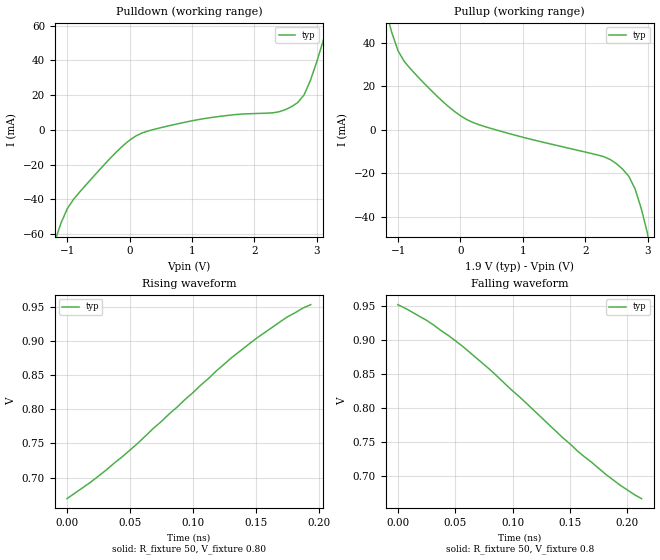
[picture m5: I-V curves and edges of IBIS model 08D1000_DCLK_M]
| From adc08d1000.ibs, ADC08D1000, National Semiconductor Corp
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[Model]   08D1000_DCLK_M
Model_type Output
Polarity Inverting
Vref=0.80
Vmeas=0.80
Rref=50   | 100 Ohms Across Outputs OUTP and OUTM
Cref=5p
|   TYP   MIN   MAX
C_comp   1.5p   1.5p   1.5p
[Temperature Range] 25   85   -40
[Voltage Range]   1.90   1.80   2.00
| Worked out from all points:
|   slope of the pulldown table from 0 to 0.285 V, typ, clamps not added: 55.2 ohm
|   slope of the pullup table from 0 to 0.285 V, typ, clamps not added: 71.5 ohm
|   falling waveform, R_fixture 50, V_fixture 0.8: 20-80 % time 113ps typ, NA min, NA max; typ from 0.952 V to 0.666 V
|   rising waveform, R_fixture 50, V_fixture 0.80: 20-80 % time 104ps typ, NA min, NA max; typ from 0.669 V to 0.953 V
[Pullup]
|Vtable   I(typ)   I(min)   I(max)
-1.9V     495.4mA    NA         NA
-1.2V     54.99mA    NA         NA
-1.1V     44.5mA     NA         NA
-1V       36.18mA    NA         NA
-800mV    27.93mA    NA         NA
-300mV    13.4mA     NA         NA
100mV     4.739mA    NA         NA
2.5V      -15.49mA   NA         NA
2.7V      -21.31mA   NA         NA
2.8V      -27.03mA   NA         NA
3V        -47.49mA   NA         NA
3.8V      -638.1mA   NA         NA
[Pulldown]
|V(pulldown)   I(typ)   I(min)   I(max)
-1.9V     -644.8mA   NA         NA
-1.2V     -64.35mA   NA         NA
-1V       -45.47mA   NA         NA
-800mV    -35.81mA   NA         NA
-200mV    -12.33mA   NA         NA
200mV     -1.805mA   NA         NA
1.1V      5.884mA    NA         NA
2.3V      9.828mA    NA         NA
2.6V      13.43mA    NA         NA
2.8V      20.25mA    NA         NA
3.2V      63.31mA    NA         NA
3.8V      497.3mA    NA         NA
[Ramp]
|   TYP   MIN   MAX
dV/dt_r   164mv/.096ns   NA   NA
dV/dt_f   164mv/.105ns   NA   NA
R_load=50
[Falling Waveform]
R_fixture=50
V_fixture=0.8
|Time   V(typ)   V(min)   V(max)
0s        952mV      NA         NA
25ps      929mV      NA         NA
56.2ps    891mV      NA         NA
81.2ps    855mV      NA         NA
156.2ps   737mV      NA         NA
181.2ps   702mV      NA         NA
193.7ps   686mV      NA         NA
212.5ps   666mV      NA         NA
[Rising Waveform]
R_fixture=50
V_fixture=0.80
|Time   V(typ)   V(min)   V(max)
0s        669mV      NA         NA
18.7ps    693mV      NA         NA
43.7ps    730mV      NA         NA
56.2ps    750mV      NA         NA
68.7ps    772mV      NA         NA
131.2ps   876mV      NA         NA
150ps     903mV      NA         NA
175ps     935mV      NA         NA
187.5ps   948mV      NA         NA
193.7ps   953mV      NA         NA
